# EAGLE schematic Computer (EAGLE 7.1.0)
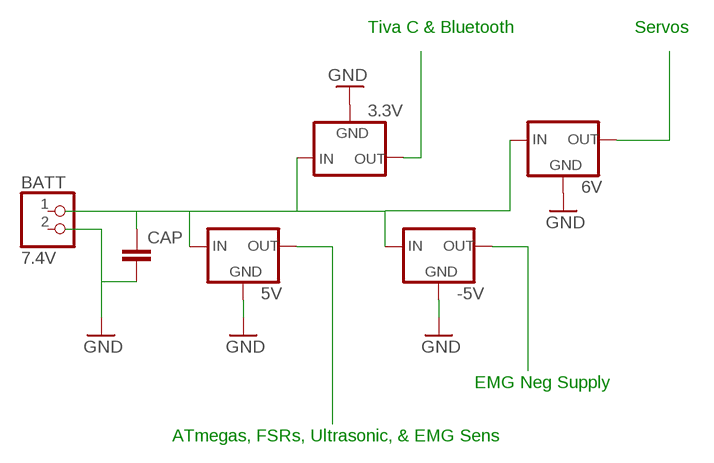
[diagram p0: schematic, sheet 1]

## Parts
3.3V  V_REG_MIC2920  [SOT223]
5V  V_REG_MIC2920  [SOT223]
6V  V_REG_MIC2920  [SOT223]
-5V  V_REG_MIC2920  [SOT223]
BATT  7.4V  PINHD-1X2/90  [1X02/90]
CAP  CAPEZ  [CAP-PTH-SMALLEZ]

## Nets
GND: 3.3V.2(GND) 5V.2(GND) 6V.2(GND) -5V.2(GND) CAP.2
N$1: 3.3V.3(OUT)
N$2: 3.3V.1(IN) 5V.1(IN) 6V.1(IN) -5V.1(IN) CAP.1
N$3: 5V.3(OUT)
N$4: 6V.3(OUT)
N$5: -5V.3(OUT)
Unconnected: BATT.1 BATT.2

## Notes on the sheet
- Tiva C & Bluetooth | Servos
- EMG Neg Supply
- ATmegas, FSRs, Ultrasonic, & EMG Sens

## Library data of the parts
3.3V 5V 6V -5V = SparkFun-PowerIC:V_REG_MIC2920: MIC2920A (http://www.micrel.com/_PDF/mic2920.pdf) - 400mA output LDO Regulator
BATT = pinhead:PINHD-1X2: PIN HEADER
CAP = SparkFun-Passives:CAP: Capacitor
